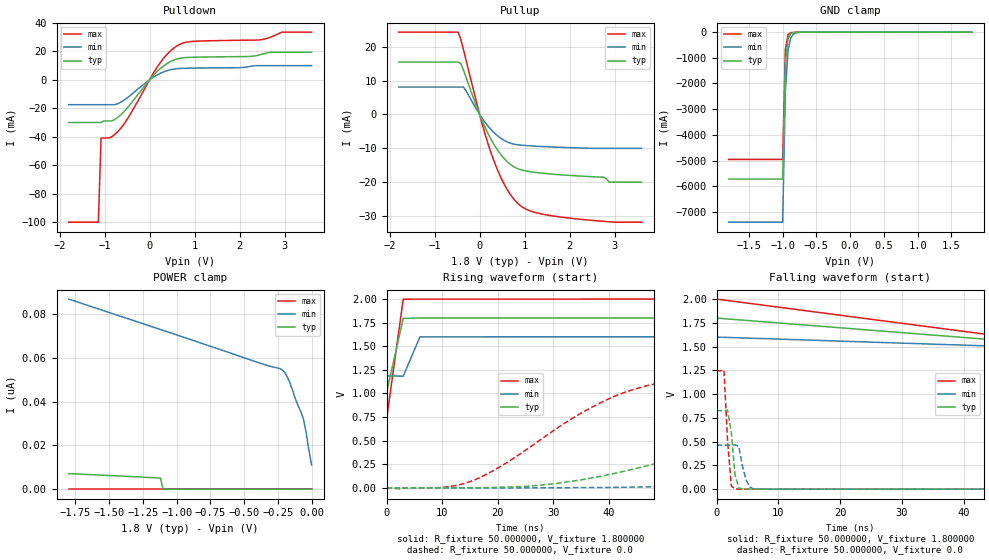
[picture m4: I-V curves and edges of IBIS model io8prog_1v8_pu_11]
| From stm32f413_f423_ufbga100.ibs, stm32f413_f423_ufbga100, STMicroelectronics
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|   Model io8prog_1v8_pu_11
[Model]  io8prog_1v8_pu_11
Model_type I/O
Polarity   Non-Inverting
Enable   Active-Low
Vinl =   0.540000V
Vinh =   1.260000V
Vmeas =  0.900000V
Cref =   100.000000pF
Rref =   1.000000k
Vref =   1.800000V
C_comp   2.595400pF   2.437600pF   2.808600pF
[Temperature Range]   25.000000   0.125000k   -40.000000
[Pullup Reference]   1.800000V   1.600000V   2.000000V
[Pulldown Reference]   0.0V   0.0V   0.0V
[POWER Clamp Reference]   1.800000V   1.600000V   2.000000V
[GND Clamp Reference]   0.0V   0.0V   0.0V
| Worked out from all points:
|   slope of the pulldown table from 0 to 0.27 V, typ, clamps not added: 31 ohm
|   slope of the pullup table from 0 to 0.27 V, typ, clamps not added: 34.9 ohm
|   GND clamp passes 1 mA (typ) near -0.57 V on its own axis
|   rising waveform, R_fixture 50.000000, V_fixture 1.800000: 20-80 % time 1.81ns typ, 1.79ns min, 1.8ns max; typ from 1.01 V to 1.8 V
|   rising waveform, R_fixture 50.000000, V_fixture 0.0: 20-80 % time 42.7ns typ, 82.3ns min, 21ns max; typ from 0 V to 0.826 V
|   falling waveform, R_fixture 50.000000, V_fixture 1.800000: 20-80 % time 93.1ns typ, 132ns min, 90.3ns max; typ from 1.8 V to 1.01 V
|   falling waveform, R_fixture 50.000000, V_fixture 0.0: 20-80 % time 754ps typ, 980ps min, 714ps max; typ from 0.826 V to 0 V
[Pulldown]
|Voltage   I(typ)   I(min)   I(max)
-1.8V     -30mA      -17.52mA   -100mA
-1.14V    -30mA      -17.52mA   -100mA
-1.08V    -30mA      -17.52mA   -40.9mA
-840mV    -28.88mA   -17.52mA   -39.94mA
-600mV    -23.35mA   -14.94mA   -32.45mA
180mV     6.236mA    3.598mA    9.492mA
540mV     13.85mA    7.499mA    22.29mA
720mV     15.32mA    8.029mA    25.55mA
900mV     15.74mA    8.167mA    26.76mA
2.46V     17.56mA    9.912mA    28.02mA
2.94V     19.29mA    9.912mA    33.46mA
3.6V      19.29mA    9.912mA    33.46mA
[Pullup]
|Voltage   I(typ)   I(min)   I(max)
-1.8V     15.46mA    8.103mA    24.33mA
-480mV    15.46mA    8.103mA    24.33mA
-360mV    13.15mA    8.103mA    19.18mA
60mV      -1.95mA    -1.198mA   -2.977mA
300mV     -8.441mA   -5.092mA   -13.07mA
600mV     -13.78mA   -8.025mA   -21.88mA
900mV     -16.27mA   -9.02mA    -26.86mA
1.2V      -17.03mA   -9.318mA   -28.8mA
1.74V     -17.75mA   -9.658mA   -30.18mA
2.76V     -18.51mA   -10mA      -31.55mA
2.88V     -20mA      -10mA      -31.68mA
3.6V      -20mA      -10mA      -31.8mA
[GND_clamp]
|Voltage   I(typ)   I(min)   I(max)
-1.8V     -5.722A    -7.401A    -4.956A
-1V       -5.722A    -7.401A    -4.956A
-960mV    -1.203A    -2.294A    -680.3mA
-920mV    -260.8mA   -717.4mA   -103.7mA
-880mV    -62.26mA   -228.9mA   -23.84mA
-840mV    -19.05mA   -76.32mA   -11.31mA
-760mV    -5.573mA   -11.66mA   -6.2mA
-640mV    -2.048mA   -2.413mA   -2.197mA
1.8V      0A         0A         0A
[POWER_clamp]
|Voltage   I(typ)   I(min)   I(max)
-1.8V     7.116nA    87.04nA    0A
-1.12V    5.066nA    73.1nA     0A
-1.1V     0A         72.68nA    0A
-220mV    0A         54.75nA    0A
-200mV    0A         53.5nA     0A
-180mV    0A         51.44nA    0A
-160mV    0A         48.56nA    0A
-120mV    0A         41.39nA    0A
-60mV     0A         32.03nA    0A
-40mV     0A         25.87nA    0A
-20mV     0A         17.74nA    0A
0V        0A         11.07nA    0A
[Ramp]
| variable   typ   min   max
dV/dt_r  0.49566/42.66378n   0.27796/83.67398n   0.74712/20.99695n
dV/dt_f  0.47520/41.50240n   0.24780/72.61905n   0.76706/23.28960n
R_load = 50.000000
[Rising Waveform]
R_fixture= 50.000000
V_fixture= 1.800000
V_fixture_min= 1.600000
V_fixture_max= 2.000000
|time   V(typ)   V(min)   V(max)
0s        1.008V     1.187V     721.6mV
3.003ns   1.794V     1.183V     1.998V
6.006ns   1.8V       1.599V     1.999V
297.3ns   1.8V       1.6V       2V
[Rising Waveform]
R_fixture= 50.000000
V_fixture= 0.0
V_fixture_min= 0.0
V_fixture_max= 0.0
|time   V(typ)   V(min)   V(max)
0s        3.541nV    238.4nV    1.408nV
10.21ns   -99.73uV   -45.35uV   5.443mV
15.62ns   1.701mV    -33.85uV   78.93mV
39.04ns   129.8mV    4.509mV    918mV
46.85ns   234.5mV    10.89mV    1.083V
56.46ns   369.1mV    19.76mV    1.177V
79.28ns   624.3mV    80.37mV    1.233V
115.3ns   782.2mV    223.5mV    1.244V
192.2ns   823.6mV    414.1mV    1.245V
299.1ns   826.1mV    463.3mV    1.245V
[Falling Waveform]
R_fixture= 50.000000
V_fixture= 1.800000
V_fixture_min= 1.600000
V_fixture_max= 2.000000
|time   V(typ)   V(min)   V(max)
0s        1.8V       1.6V       2V
150.2ns   1.033V     1.282V     723.9mV
300.3ns   1.008V     1.194V     721.6mV
450.5ns   1.008V     1.188V     721.6mV
14.86us   1.008V     1.187V     721.6mV
[Falling Waveform]
R_fixture= 50.000000
V_fixture= 0.0
V_fixture_min= 0.0
V_fixture_max= 0.0
|time   V(typ)   V(min)   V(max)
0s        826.1mV    463.3mV    1.245V
1.201ns   825.8mV    463.3mV    1.254V
1.802ns   831.3mV    463.3mV    492.6mV
2.402ns   589mV      462.6mV    30.52mV
3.003ns   147mV      465.9mV    2.705mV
3.604ns   13.54mV    450mV      738.7uV
4.805ns   651.4uV    93.32mV    376.7uV
5.405ns   359uV      21.23mV    297.7uV
6.607ns   203.1uV    1.205mV    212.9uV
299.1ns   3.541nV    238.4nV    1.408nV
